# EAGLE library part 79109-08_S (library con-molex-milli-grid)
RECEPTACAL
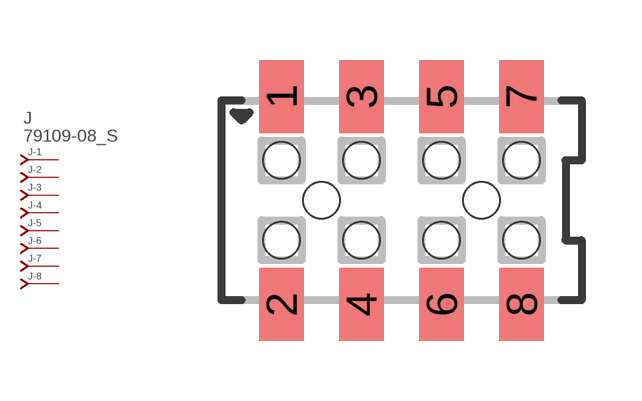
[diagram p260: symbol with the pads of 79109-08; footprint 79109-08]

Designator prefix J; gates -1=J-NV -2=J-N -3=J-N -4=J-N -5=J-N -6=J-N -7=J-N -8=J-N

## 79109-08_S  [79109-08]
1  -1:J  pas
2  -2:J  pas
3  -3:J  pas
4  -4:J  pas
5  -5:J  pas
6  -6:J  pas
7  -7:J  pas
8  -8:J  pas

## Footprint 79109-08 (pad centres in mm)
RECEPTACAL SMD Dual Row, Vertical, Pass-Thru
smd 1.12 x 1.83: 1 -3,2.6; 2 -3,-2.6; 3 -1,2.6; 4 -1,-2.6; 5 1,2.6; 6 1,-2.6; 7 3,2.6; 8 3,-2.6
hole 0.914 at -2,0
hole 0.914 at -3,1
hole 0.914 at -3,-1
hole 0.914 at -1,-1
hole 0.914 at -1,1
hole 0.914 at 1,-1
hole 0.914 at 1,1
hole 0.914 at 2,0
hole 0.914 at 3,1
hole 0.914 at 3,-1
